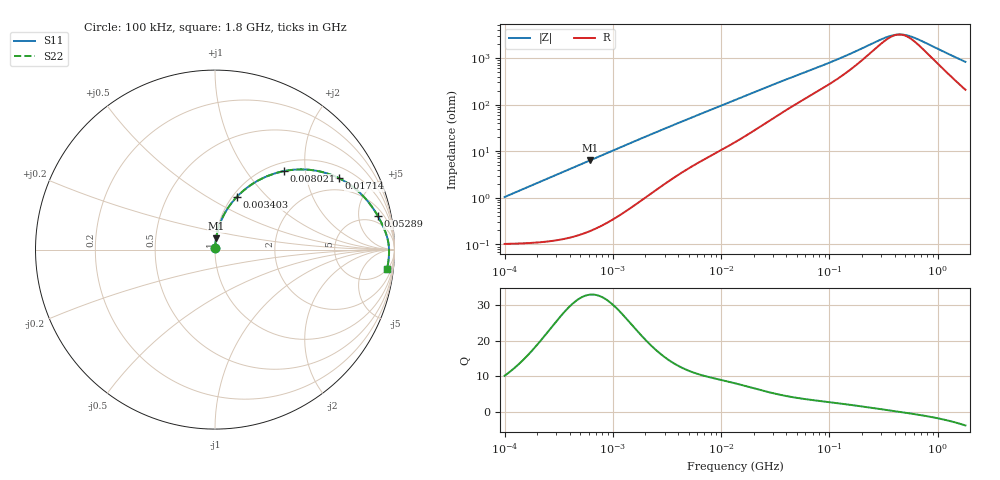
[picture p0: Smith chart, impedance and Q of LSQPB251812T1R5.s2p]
! LSQPB251812T1R5  S-PARAMETER MODEL  ( General Type )
! Model Generated by TAIYO YUDEN Corporation (http://www.ty-top.com)
! Version 2.0
! TAIYO YUDEN Control No. 100810NF18SB-HKC
! Copyright(c) 2007 TAIYO YUDEN CO.,LTD. All Rights Reserved.
! Product Description (link to TY-COMPAS)
! https://ds.yuden.co.jp/TYCOMPAS/or/detail?pn=LSQPB251812T1R5M&u=M
! Products Name : Inductors
! Characteristics :
!  Inductance : 1.5 uH , SRF(min) : 100 MHz , DC Resistance(max) : 0.13 Ohm
!  Rated Current : Saturation :1200 mA , Temp Rise : 920 mA (40 degC)
!  Case Size : 2.5 x 1.8 / 0.098 x 0.071 [mm/inch] , Thickness : 1.2 / 0.048 [mm/inch]
!  (Conditions: Temperature = 25 degC , DC Bias Current/Voltage = 0A / 0V)
! External Node Assignments :
!  1  o---GGG---o  2
! GND o---------o GND
! Frequency Range : 0.1MHz  -  1800MHz  [ 402 STEP ]
# MHz S RI R 50
! Freq[MHz].  S11 Real  S11 Imag  S21 Real  S21 Imag  S12 Real  S12 Imag  S22 Real  S22 Imag
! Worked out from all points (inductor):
!   401 points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, 100 kHz to 1.8 GHz, reference 50 ohm
!   read as one part in series: L = 1.65 uH near 105 kHz
!   highest Q = 32.9 at 612.7 kHz (marker M1), where L = 1.65 uH
!   self-resonance near 438.8 MHz
!   S11 on the Smith chart (normalised r, x): 100 kHz: 1.00, +0.02; 3.403 MHz: 1.05, +0.69; 8.021 MHz: 1.16, +1.54; 17.14 MHz: 1.44, +3.14; 52.89 MHz: 3.28, +8.63; 1.8 GHz: 5, -16
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0.1  0.00113 0.0103  0.9989 -0.0103  0.9989 -0.0103  0.00113 0.0103
0.516129  0.00449 0.0531  0.9955 -0.0531  0.9955 -0.0531  0.00449 0.0531
0.612668  0.00591 0.0629  0.9941 -0.0629  0.9941 -0.0629  0.00591 0.0629
1.309209  0.0227 0.1313  0.9773 -0.1313  0.9773 -0.1313  0.0227 0.1313
2.66389  0.0813 0.2449  0.9187 -0.2449  0.9187 -0.2449  0.0813 0.2449
3.403283  0.122 0.294  0.878 -0.294  0.878 -0.294  0.122 0.294
5.161158  0.2263 0.3769  0.7737 -0.3769  0.7737 -0.3769  0.2263 0.3769
8.02111  0.3859 0.4376  0.6141 -0.4376  0.6141 -0.4376  0.3859 0.4376
10.50158  0.4991 0.4464  0.5009 -0.4464  0.5009 -0.4464  0.4991 0.4464
13.41641  0.6009 0.4313  0.3991 -0.4313  0.3991 -0.4313  0.6009 0.4313
17.14029  0.692 0.3972  0.308 -0.3972  0.308 -0.3972  0.692 0.3972
21.89777  0.7665 0.351  0.2335 -0.351  0.2335 -0.351  0.7665 0.351
28.66948  0.8279 0.2958  0.1721 -0.2958  0.1721 -0.2958  0.8279 0.2958
52.8901  0.9078 0.1861  0.0922 -0.1861  0.0922 -0.1861  0.9078 0.1861
69.24595  0.9275 0.1489  0.0725 -0.1489  0.0725 -0.1489  0.9275 0.1489
134.1607  0.956 0.0793  0.044 -0.0793  0.044 -0.0793  0.956 0.0793
293.7968  0.968 0.0232  0.032 -0.0232  0.032 -0.0232  0.968 0.0232
357.3983  0.9691 0.0117  0.0309 -0.0117  0.0309 -0.0117  0.9691 0.0117
445.5497  0.9697 -0.000866  0.0303 0.000866  0.0303 0.000866  0.9697 -0.000866
503.6016  0.9698 -0.00785  0.0302 0.00785  0.0302 0.00785  0.9698 -0.00785
569.2172  0.9698 -0.015  0.0302 0.015  0.0302 0.015  0.9698 -0.015
1800  0.9582 -0.1088  0.0418 0.1088  0.0418 0.1088  0.9582 -0.1088
